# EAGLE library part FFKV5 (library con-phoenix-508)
PHOENIX
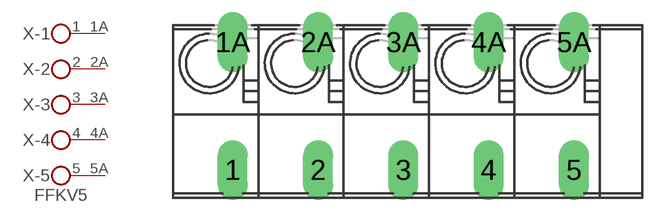
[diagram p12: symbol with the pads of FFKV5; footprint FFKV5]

Designator prefix X; gates -1=KL2 -2=KL2 -3=KL2 -4=KL2 -5=KL2V

## FFKV5 (OC_FARNELL: unknown; OC_NEWARK: unknown)  [FFKV5]
1  -1:1  pas
1A  -1:2  pas
2  -2:1  pas
2A  -2:2  pas
3  -3:1  pas
3A  -3:2  pas
4  -4:1  pas
4A  -4:2  pas
5  -5:1  pas
5A  -5:2  pas

## Footprint FFKV5 (pad centres in mm)
PHOENIX
drill 1.194 long: 1 -10.16,-3.81; 1A -10.16,3.81; 2 -5.08,-3.81; 2A -5.08,3.81; 3 0,-3.81; 3A 0,3.81; 4 5.08,-3.81; 4A 5.08,3.81; 5 10.16,-3.81; 5A 10.16,3.81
